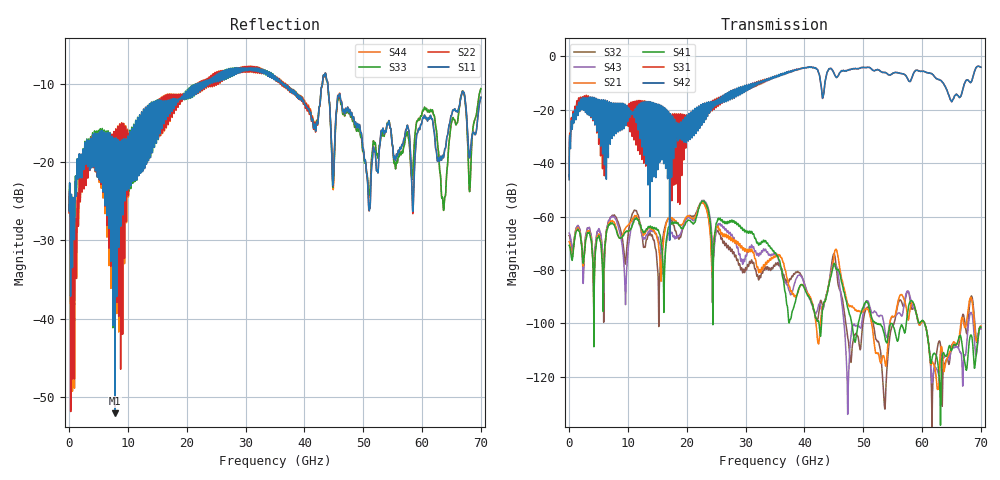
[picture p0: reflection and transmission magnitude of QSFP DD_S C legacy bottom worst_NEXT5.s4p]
! AWR Design Environment (8415) Thu Dec 20 15:47:00 2018
! Document = 'CHANNEL TEST'
! nPorts: 4, nXvals: 7001
# HZ S DB R 50
!Freq DBS11 AngS11 DBS12 AngS12 DBS13 AngS13 DBS14 AngS14
!	DBS21 AngS21 DBS22 AngS22 DBS23 AngS23 DBS24 AngS24
!	DBS31 AngS31 DBS32 AngS32 DBS33 AngS33 DBS34 AngS34
!	DBS41 AngS41 DBS42 AngS42 DBS43 AngS43 DBS44 AngS44
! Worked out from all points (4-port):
!   7000 points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, 10 MHz to 70 GHz, reference 50 ohm
!   strongest paths, dB at 10 MHz, 17.51 GHz, 35.01 GHz, 52.51 GHz, 70 GHz:
!     S42: -46.2, -25.1, -7.4, -5.0, -4.0
!     S31: -45.2, -30.1, -7.6, -5.0, -4.0
!     S41: -70.8, -62.1, -73.7, -100.1, -101.4
!     S21: -69.4, -60.4, -75.1, -111.1, -100.9
!     S43: -66.2, -65.9, -74.1, -97.0, -102.1
!     S32: -67.1, -61.5, -78.3, -106.7, -101.7
!   lowest |S11| = -52.1 dB at 7.78 GHz (marker M1), VSWR 1.00, Z = 49.9 - j0.242 ohm
!   |S11| at or under -10 dB: start of sweep to 21.78 GHz; 36.28 GHz to 43.07 GHz (6.789 GHz wide, 17.1 % of centre); 43.97 GHz to end of sweep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
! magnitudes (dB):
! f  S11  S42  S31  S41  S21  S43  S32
! 10 MHz  -26.3  -46.2  -45.2  -70.8  -69.4  -66.2  -67.1
! 1.65 GHz  -19.9  -17.2  -15.5  -65.4  -64.8  -64.0  -64.0
! 7.78 GHz  -52.1  -17.9  -18.9  -63.7  -62.7  -60.4  -59.6
! 9.59 GHz  -17.7  -23.0  -19.4  -65.9  -64.3  -92.7  -77.5
! 22.8 GHz  -9.7  -19.4  -19.9  -54.3  -55.0  -54.0  -54.8
! 29.48 GHz  -8.1  -11.5  -12.1  -64.9  -72.4  -77.8  -81.0
! 70 GHz  -11.8  -4.0  -4.0  -101.4  -100.9  -102.1  -101.7
